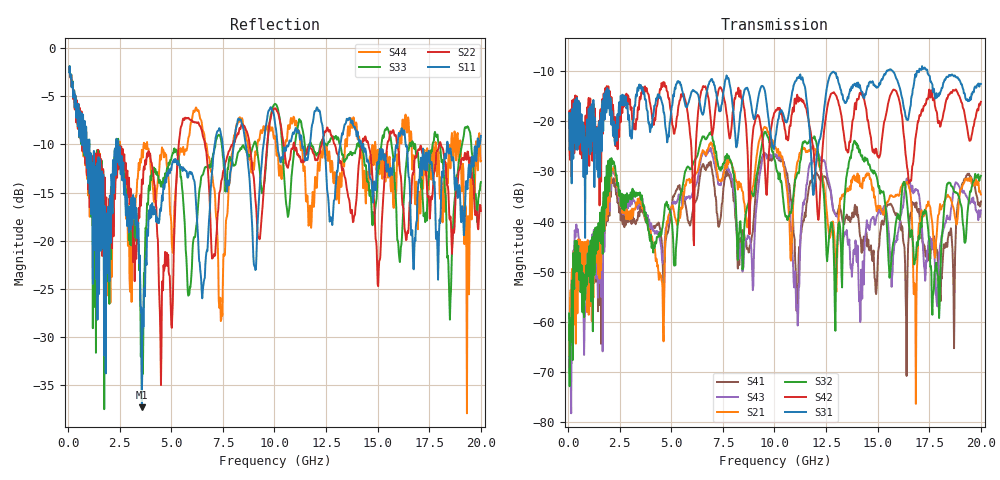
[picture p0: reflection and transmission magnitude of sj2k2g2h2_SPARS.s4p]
! FILE: E:\users\goganessyan\GBX_Backplane\FR408_backplane\1m_OUTBOUND_NEXT\sj2k2g2h2_SPARS.s4p
# MHZ S RI R 50.00
! FREQ  S11  S12  S13  S14
!  S21  S22  S23  S24
!  S31  S32  S33  S34
!  S41  S42  S43  S44
!  REAL  IMAG  REAL  IMAG  REAL  IMAG  REAL  IMAG
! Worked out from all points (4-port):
!   799 points, 50 MHz to 20 GHz, reference 50 ohm
!   strongest paths, dB at 50 MHz, 5.025 GHz, 10.03 GHz, 15.03 GHz, 20 GHz:
!     S31: -18.4, -17.1, -23.9, -13.2, -12.6
!     S42: -18.1, -19.8, -18.2, -27.0, -16.2
!     S32: -58.3, -39.8, -27.9, -32.9, -30.9
!     S21: -66.5, -37.1, -25.2, -36.8, -34.6
!     S43: -67.2, -37.2, -26.7, -38.1, -37.8
!     S41: -60.7, -36.9, -27.0, -45.9, -36.0
!   lowest |S11| = -37.3 dB at 3.575 GHz (marker M1), VSWR 1.03, Z = 48.7 + j0.353 ohm
!   |S11| at or under -10 dB: 2.43 GHz to 7.101 GHz (4.671 GHz wide, 98 % of centre); 14.3 GHz to 15.97 GHz (1.663 GHz wide, 11 % of centre); 16.35 GHz to 18.37 GHz (2.011 GHz wide, 11.6 % of centre)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
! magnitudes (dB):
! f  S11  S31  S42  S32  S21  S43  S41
! 50 MHz  -2.5  -18.4  -18.1  -58.3  -66.5  -67.2  -60.7
! 400 MHz  -7.2  -21.7  -16.0  -43.8  -45.1  -40.6  -44.5
! 3.575 GHz  -37.3  -13.9  -14.5  -34.8  -36.3  -35.9  -37.2
! 12.95 GHz  -14.6  -10.6  -14.8  -61.7  -48.3  -38.5  -38.4
! 13.9 GHz  -8.2  -12.7  -16.4  -24.1  -31.7  -46.5  -36.7
! 17.68 GHz  -13.0  -14.2  -15.9  -54.8  -42.0  -44.9  -45.1
! 20 GHz  -9.1  -12.6  -16.2  -30.9  -34.6  -37.8  -36.0
